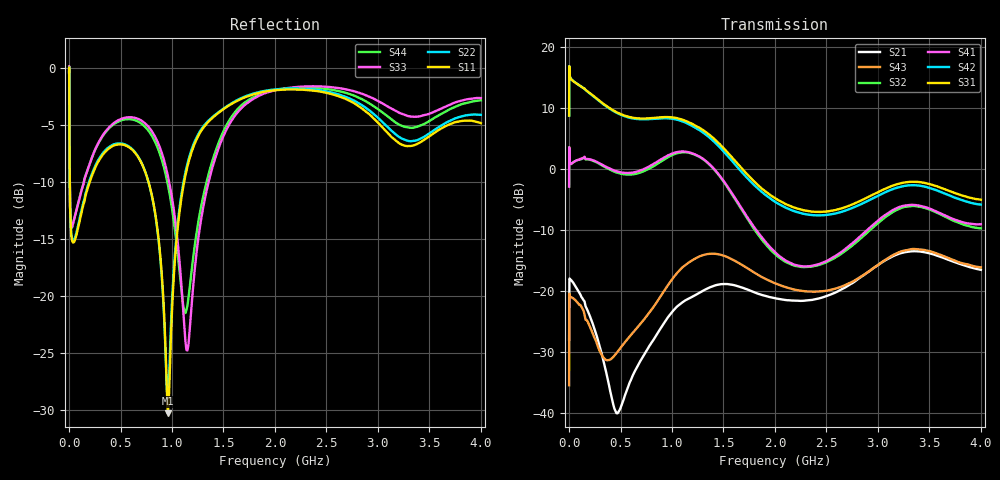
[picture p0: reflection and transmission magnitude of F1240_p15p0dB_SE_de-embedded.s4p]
! Integrated Device Technology
! Corporate Headquarters
! 6024 Silver Creek Valley Road
! San Jose, CA 95138  USA
! Phone:  1-408-284-8200
! Toll Free:  1-800-223-1366
! Webpage:  http://www.idt.com/
! Timing and RF Division
! 515 Groton Road, Suite 102
! Westford, MA 01886-6024
! Device:  F1240
! Description: Dual Intermediate Frequency Digital Variable Gain Amplifier
! Frequency:  10.0 -  500.00 MHz
! Package:  5x5 mm QFN Plastic Package: 32 pin
! Ports:  8 RF, 20 DC
!  Pin  1  = GA3 / Data  Pin 17  = RF OUT_B+
!  Pin  2  = GA4 / CLK  Pin 18  = RF OUT_B-
!  Pin  3  = GA5  Pin 19  = STBY_B
!  Pin  4  = VMODE  Pin 20  = Ground
!  Pin  5  = No Connect  Pin 21  = Ground
!  Pin  6  = GB5  Pin 22  = STB_A
!  Pin  7  = GB4  Pin 23  = RF OUT_A-  = Port 4
!  Pin  8  = GB3  Pin 24  = RF OUT_A+  = Port 3
!  Pin  9  = GB2  Pin 25  = GA0
!  Pin 10  = GB1  Pin 26  = ISET_A
!  Pin 11  = RF IN_B+  Pin 27  = VCC
!  Pin 12  = RF IN_B-  Pin 28  = Ground
!  Pin 13  = Ground  Pin 29  = RF IN_A-  = Port 2
!  Pin 14  = VCC  Pin 30  = RF IN_A+  = Port 1
!  Pin 15  = ISET_B  Pin 31  = GA1
!  Pin 16  = GB0  Pin 32  = GA2 / CSb
! Gain  = +19.5 dB
! State  = 1
! Voltage  = +5.00 V
! Current  = 85.292 mA (one channel only)
! Temperture  =  +25 C
! Test Date  =  2017-10-18
! Board  =  EB4031
! Data:  The device was measured on a custom evaluation board which has
!  individual transmission lines to the RF pins.  Data was collected
!  using a calibrated network analyzer.  The evaluation board was
!  de-embedded using Automatic Fixture Removal.
!  The reference plane is the edge of the package pin.
!  Only Channel A was measured.
!  This data is in single-ended operation.  If your needs are balanced
!  or differential S-parameters then this file needs to be used a
!  linear simulator.
! File Date:  2017-11-10  MJV
! Note:
!  Integrated Device Technology supplies this data as a sample of measured
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# Hz S dB R 100
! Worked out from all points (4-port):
!   410 points, 500 kHz to 4 GHz, reference 100 ohm
!   strongest paths, dB at 500 kHz, 930 MHz, 1.96 GHz, 2.98 GHz, 4 GHz:
!     S31: 8.8, 8.5, -4.3, -3.9, -5.0
!     S42: 8.8, 8.4, -4.9, -4.6, -5.8
!     S41: -2.9, 2.0, -13.0, -8.8, -9.1
!     S32: -2.9, 1.6, -13.3, -9.2, -9.7
!     S43: -35.5, -19.8, -18.5, -16.0, -16.2
!     S21: -28.1, -25.1, -21.1, -16.0, -16.6
!   lowest |S11| = -30.3 dB at 960 MHz (marker M1), VSWR 1.06, Z = 105 + j3.42 ohm
!   |S11| at or under -10 dB: 7.243 MHz to 200.6 MHz (193.4 MHz wide, 186 % of centre); 771.6 MHz to 1.117 GHz (345.8 MHz wide, 36.6 % of centre)
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500000  -0.35 -6.2  -28.07 4.7  -27.37 76.0  -60.45 67.7
        -28.07 4.1  -0.35 -6.1  -60.28 62.7  -27.37 77.3
        8.79 -105.3  -2.86 72.0  -0.45 1.1  -35.59 -151.5
        -2.88 73.1  8.76 -104.1  -35.53 -151.4  -0.45 3.4
3000000  -4.50 -53.5  -18.36 16.8  -19.02 14.4  -40.72 58.2
         -18.34 16.8  -4.46 -53.6  -40.72 58.0  -19.03 14.6
         16.43 -171.8  2.17 -4.1  -4.10 -48.9  -20.52 38.9
         2.17 -4.0  16.42 -171.6  -20.49 38.8  -4.16 -48.7
2e8  -10.02 -114.9  -23.99 -101.3  -21.79 -51.8  -33.98 10.5
     -24.06 -100.1  -9.83 -116.6  -33.97 10.7  -21.81 -51.8
     12.50 109.2  1.53 -52.5  -8.42 -80.4  -25.21 -115.1
     1.61 -52.6  12.46 108.4  -25.80 -113.4  -8.41 -79.8
5.4e8  -6.77 -173.3  -37.04 53.0  -23.58 -107.9  -27.97 -58.0
       -37.32 41.7  -6.69 -174.6  -28.12 -56.6  -23.73 -108.2
       8.78 24.8  -0.88 -128.6  -4.37 -151.0  -29.33 61.2
       -0.63 -129.7  8.67 23.7  -28.49 43.0  -4.51 -150.8
9.6e8  -30.30 32.1  -22.94 -53.5  -20.94 166.8  -23.33 -156.8
       -24.35 -61.9  -29.26 21.2  -23.68 -152.0  -21.37 166.2
       8.54 -77.1  1.94 140.3  -9.47 144.0  -19.62 -36.1
       2.24 135.6  8.34 -78.9  -19.09 -53.6  -10.25 147.5
1.52e9  -3.48 -145.8  -18.65 156.2  -26.92 35.9  -25.42 69.1
        -18.89 160.8  -3.43 -146.1  -25.33 75.0  -28.20 34.3
        3.09 122.1  -2.54 -43.8  -5.57 -127.8  -14.47 149.0
        -2.40 -48.8  2.55 120.7  -14.34 142.7  -5.18 -131.3
4e9  -4.84 -156.5  -16.59 60.6  -21.59 -43.0  -19.64 -48.3
     -16.55 60.0  -4.11 -150.6  -22.04 -29.6  -25.12 -29.5
     -5.03 7.6  -9.75 -121.7  -2.64 -136.5  -15.29 90.9
     -9.06 -132.6  -5.84 16.8  -16.16 63.6  -2.83 -141.9
